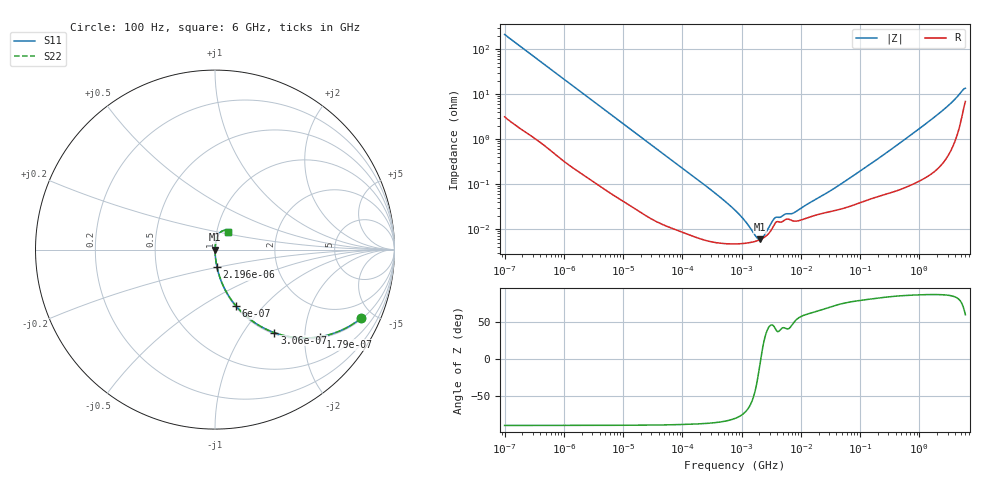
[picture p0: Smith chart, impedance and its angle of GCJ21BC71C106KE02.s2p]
!Murata Part Number: GCJ21BC71C106KE02
!These Parameters are Measured in Series Mode Connection
!Data Generated on Mar 13, 2026
!  o--ll--o
!Port1  Port2
!  o------o
!Operation Temp=25[degC], DC Bias Voltage=0[V]
!Freq. Start=100[Hz] Stop=6[GHz] 401[Steps]
# Hz S RI R 50
!Freq.(Hz) S11(Real) S11(Imag) S21(Real) S21(Imag) S12(Real) S12(Imag) S22(Real) S22(Imag)
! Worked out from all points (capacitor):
!   401 points, 100 Hz to 6 GHz, reference 50 ohm
!   read as one part in series: C = 7.49 uF near 109 Hz
!   lowest |Z| = 5.88 mohm at 2.074 MHz (marker M1)
!   series resonance near 2.109 MHz, so ESL is about 760 pH
!   S11 on the Smith chart (normalised r, x): 100 Hz: 1.06, -4.24; 179 Hz: 1.04, -2.38; 306 Hz: 1.02, -1.40; 600 Hz: 1.01, -0.72; 2.196 kHz: 1.00, -0.20; 6 GHz: 1.14, +0.23
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100  0.8143 -0.3815  0.1857 0.3815  0.1857 0.3815  0.8143 -0.3815
179  0.5848 -0.4854  0.4152 0.4854  0.4152 0.4854  0.5848 -0.4854
306  0.3306 -0.4627  0.6694 0.4627  0.6694 0.4627  0.3306 -0.4627
600  0.1183 -0.3154  0.8817 0.3154  0.8817 0.3154  0.1183 -0.3154
981  0.0493 -0.2092  0.9507 0.2092  0.9507 0.2092  0.0493 -0.2092
2008  0.0133 -0.1069  0.9867 0.1069  0.9867 0.1069  0.0133 -0.1069
2196  0.0113 -0.098  0.9887 0.098  0.9887 0.098  0.0113 -0.098
6728  0.00165 -0.0327  0.9984 0.0327  0.9984 0.0327  0.00165 -0.0327
40335  0.000169 -0.00557  0.9998 0.00557  0.9998 0.00557  0.000169 -0.00557
316350  5.24e-05 -0.000713  0.9999 0.000713  0.9999 0.000713  5.24e-05 -0.000713
774597  4.69e-05 -0.000259  1 0.000259  1 0.000259  4.69e-05 -0.000259
1449809  5.07e-05 -8.53e-05  0.9999 8.53e-05  0.9999 8.53e-05  5.07e-05 -8.53e-05
2074311  5.87e-05 -3.7e-06  0.9999 3.7e-06  0.9999 3.7e-06  5.87e-05 -3.7e-06
2713602  7.39e-05 5.92e-05  0.9999 -5.92e-05  0.9999 -5.92e-05  7.39e-05 5.92e-05
3712478  0.000137 0.000118  0.9999 -0.000118  0.9999 -0.000118  0.000137 0.000118
7599586  0.000151 0.000173  0.9998 -0.000173  0.9998 -0.000173  0.000151 0.000173
1.555665e7  0.000193 0.000366  0.9998 -0.000366  0.9998 -0.000366  0.000193 0.000366
4.556224e7  0.000275 0.000928  0.9997 -0.000928  0.9997 -0.000928  0.000275 0.000928
3.124326e8  0.000657 0.00549  0.9993 -0.00549  0.9993 -0.00549  0.000657 0.00549
2.048624e9  0.00343 0.0351  0.9966 -0.0351  0.9966 -0.0351  0.00343 0.0351
4.193612e9  0.0169 0.0795  0.9831 -0.0795  0.9831 -0.0795  0.0169 0.0795
6e9  0.0752 0.1006  0.9248 -0.1006  0.9248 -0.1006  0.0752 0.1006
